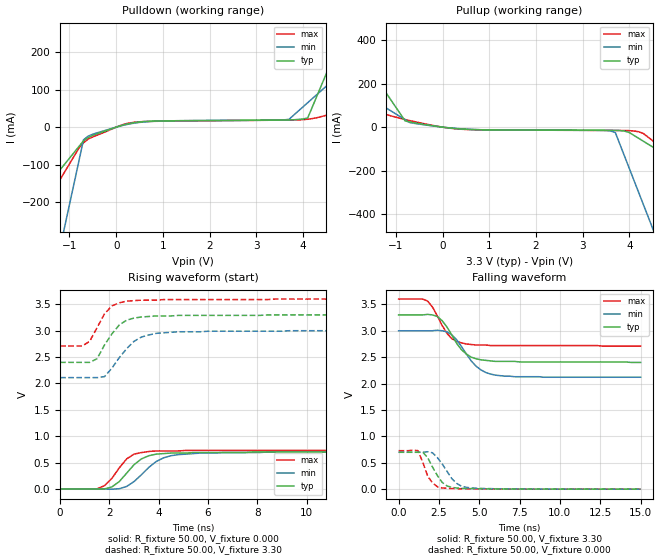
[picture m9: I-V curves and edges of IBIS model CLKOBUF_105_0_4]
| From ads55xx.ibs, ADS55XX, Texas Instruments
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|   Model CLKOBUF_105_0_4
[Model]   CLKOBUF_105_0_4
Model_type   Output
Polarity   Non-Inverting
Vmeas =   1.65V
C_comp   2pf   2pf   2pf
[Temperature Range]   50.00   0.10k   -20.00
[Voltage Range]   3.30V   3.00V   3.60V
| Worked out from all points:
|   slope of the pulldown table from 0 to 0.495 V, typ, clamps not added: 36.2 ohm
|   slope of the pullup table from 0 to 0.495 V, typ, clamps not added: 50.9 ohm
|   rising waveform, R_fixture 50.00, V_fixture 0.000: 20-80 % time 873ps typ, 1.07ns min, 764ps max; typ from 0 V to 0.7 V
|   rising waveform, R_fixture 50.00, V_fixture 3.30: 20-80 % time 806ps typ, 986ps min, 702ps max; typ from 2.4 V to 3.3 V
|   falling waveform, R_fixture 50.00, V_fixture 3.30: 20-80 % time 1.25ns typ, 1.33ns min, 1.04ns max; typ from 3.3 V to 2.4 V
|   falling waveform, R_fixture 50.00, V_fixture 0.000: 20-80 % time 808ps typ, 996ps min, 639ps max; typ from 0.7 V to 0.001 V
[Pulldown]
| voltage   I(typ)   I(min)   I(max)
-3.3V     -435.6mA   -1.525A    -575.1mA
-2.3V     -282.1mA   -951.2mA   -367.5mA
-1.9V     -220.7mA   -721.8mA   -284.5mA
-1.5V     -159.3mA   -492.4mA   -201.4mA
-1V       -82.55mA   -205.7mA   -97.63mA
-700mV    -36.5mA    -33.62mA   -41.61mA
200mV     7.4mA      6.35mA     8.74mA
3.7V      19.01mA    20.77mA    18.9mA
4.1V      24.13mA    64.93mA    21.03mA
4.9V      260.8mA    153.2mA    44.43mA
5.9V      556.6mA    263.6mA    76.63mA
6.6V      763.6mA    340.9mA    99.17mA
[Pullup]
| voltage   I(typ)   I(min)   I(max)
-3.3V     820.4mA    365.6mA    174.6mA
-2.3V     503.6mA    233.1mA    118.7mA
-2.1V     440.2mA    206.5mA    107.5mA
-800mV    28.36mA    34.15mA    34.85mA
-600mV    19.95mA    17.19mA    25.34mA
400mV     -8.46mA    -7.79mA    -9.63mA
3.6V      -14.59mA   -17.79mA   -15.28mA
3.7V      -14.79mA   -24.94mA   -15.36mA
4V        -24.95mA   -190.5mA   -16.18mA
4.2V      -51.53mA   -300.9mA   -21.09mA
4.5V      -91.4mA    -466.5mA   -62.35mA
6.6V      -370.5mA   -1.625A    -410.2mA
[Ramp]
| variable   typ   min   max
dV/dt_r   0.42/0.86n   0.42/1.04n   0.44/0.75n
dV/dt_f   0.54/1.20n   0.53/1.33n   0.53/1.01n
R_load = 50.00
[Rising Waveform]
R_fixture = 50.00
V_fixture = 0.000
V_fixture_min = 0.000
V_fixture_max = 0.000
| time   V(typ)   V(min)   V(max)
0s        33.02nV    41.91nV    67.33nV
1.5ns     -2.44mV    38.23uV    1.69mV
1.8ns     -890uV     -1.74mV    61.5mV
2.1ns     37.57mV    -4.79mV    200mV
2.7ns     300mV      47.3mV     570mV
3ns       460mV      140mV      660mV
3.6ns     630mV      410mV      710mV
4.5ns     680mV      630mV      720mV
5.7ns     690mV      680mV      730mV
15ns      700mV      700mV      730mV
[Rising Waveform]
R_fixture = 50.00
V_fixture = 3.30
V_fixture_min = 3.00
V_fixture_max = 3.60
| time   V(typ)   V(min)   V(max)
0s        2.4V       2.11V      2.71V
900ps     2.4V       2.11V      2.71V
1.2ns     2.4V       2.11V      2.8V
1.5ns     2.47V      2.11V      3.06V
1.8ns     2.73V      2.13V      3.32V
2.1ns     2.94V      2.29V      3.47V
2.7ns     3.2V       2.66V      3.56V
3.3ns     3.26V      2.88V      3.58V
4.8ns     3.29V      2.98V      3.59V
15ns      3.3V       3V         3.6V
[Falling Waveform]
R_fixture = 50.00
V_fixture = 3.30
V_fixture_min = 3.00
V_fixture_max = 3.60
| time   V(typ)   V(min)   V(max)
0s        3.3V       3V         3.6V
1.5ns     3.3V       3V         3.6V
1.8ns     3.31V      3V         3.56V
2.4ns     3.27V      3.01V      3.28V
3ns       3.07V      2.98V      2.95V
3.3ns     2.92V      2.92V      2.85V
4.2ns     2.56V      2.56V      2.75V
5.1ns     2.45V      2.26V      2.73V
6ns       2.42V      2.16V      2.72V
15ns      2.4V       2.12V      2.71V
[Falling Waveform]
R_fixture = 50.00
V_fixture = 0.000
V_fixture_min = 0.000
V_fixture_max = 0.000
| time   V(typ)   V(min)   V(max)
0s        700mV      700mV      730mV
1.2ns     700mV      700mV      730mV
1.5ns     700mV      700mV      510mV
1.8ns     600mV      710mV      250mV
2.1ns     420mV      690mV      120mV
2.7ns     130mV      480mV      24.62mV
3.3ns     35.32mV    200mV      13.44mV
3.6ns     23.76mV    110mV      10.85mV
4.2ns     13.94mV    36.12mV    7.91mV
15ns      1.32mV     1.64mV     1.38mV
